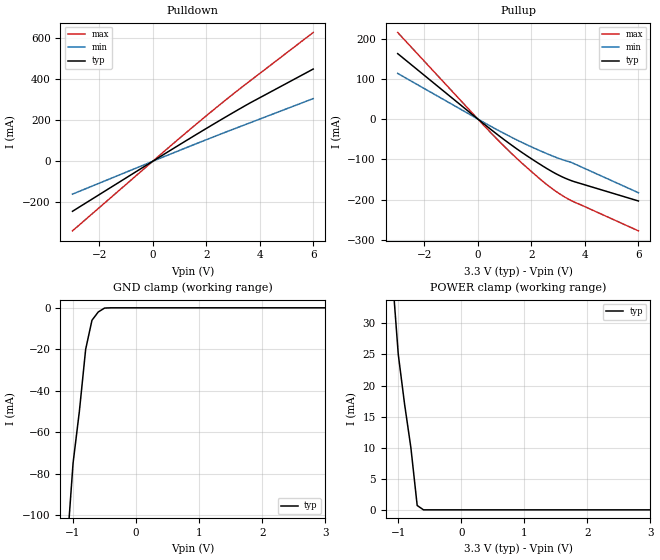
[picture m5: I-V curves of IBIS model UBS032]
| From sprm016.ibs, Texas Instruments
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[Model]   UBS032
Model_type   I/O
Polarity   Non-Inverting
| signals   A, GZ, Y1, Y2
Vinl = 0.8V
Vinh = 2.0V
Cref = 30p
Rref = 50
Vref = 1.5
Vmeas = 1.5
|   typ   min   max
C_comp   9.5590p   9.5244p   9.7951p
|   typ   min   max
[Temperature Range]   25.0   0   90
|   typ   min   max
[Voltage Range]   3.3V   3.13V   3.47V
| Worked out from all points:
|   slope of the pulldown table from 0 to 0.495 V, typ, clamps not added: 12.3 ohm
|   slope of the pullup table from 0 to 0.495 V, typ, clamps not added: 18.8 ohm
|   GND clamp passes 1 mA (typ) near -0.55 V on its own axis
|   POWER clamp passes 1 mA (typ) near -0.70 V on its own axis
[Pulldown]
|   Voltage   I(typ)   I(min)   I(max)
-3V       -243.9mA   -160.2mA   -339.3mA
500mV     40.51mA    26.57mA    56.33mA
2.1V      167.6mA    110.2mA    232.3mA
3.6V      281.7mA    185.8mA    388.3mA
6V        449.8mA    305.8mA    628.1mA
[GND_clamp]
|   Voltage   I(typ)   I(min)   I(max)
-3V       -900mA     NA         NA
-2V       -500mA     NA         NA
-1V       -75mA      NA         NA
-900mV    -50mA      NA         NA
-800mV    -20mA      NA         NA
-700mV    -6mA       NA         NA
-600mV    -2mA       NA         NA
-500mV    -120uA     NA         NA
-400mV    0A         NA         NA
3V        0A         NA         NA
[Pullup]
|   Voltage   I(typ)   I(min)   I(max)
-3V       162.6mA    113.5mA    215.1mA
600mV     -31.75mA   -22.18mA   -41.98mA
1.5V      -76.07mA   -53.22mA   -100.5mA
2.4V      -115.5mA   -80.73mA   -153.2mA
2.9V      -135.1mA   -94.54mA   -178.7mA
3.4V      -150.5mA   -105.6mA   -199.3mA
6V        -203.3mA   -182.8mA   -277.5mA
[POWER_clamp]
|   Voltage   I(typ)   I(min)   I(max)
-3V       300mA      NA         NA
-2V       160mA      NA         NA
-1V       25mA       NA         NA
-900mV    17mA       NA         NA
-800mV    10mA       NA         NA
-700mV    700uA      NA         NA
-600mV    0A         NA         NA
-500mV    0A         NA         NA
3V        0A         NA         NA
[Ramp]
|   I(typ)   I(min)   I(max)
dV/dt_r   1.501/1.270n   1.256/1.780n   1.674/0.980n
dV/dt_f   1.504/1.320n   1.273/1.950n   1.674/0.960n
